PROGRAM MAIN
VAR
	init : BOOL;
	initSubstate : InitSubstate;
	axisPowerSubstate : AxisPowerSubstate; 
	solenoindExtendSubstate : SolenoindExtendSubstate;
	isInit, hasNext, isPower, isBackToInit : BOOL;
	applicationState  : ApplicationSubstate;
	
	axisModule : AxisModule(applicationState, InitSubstate := initSubstate, AxisPowerSubstate := solenoindExtendSubstate);
	pusherModule : PusherModule(applicationState);
END_VAR

IF NOT init THEN
	applicationState.AddSubstate(initSubstate);
	applicationState.AddSubstate(solenoindExtendSubstate);
	applicationState.AddSubstate(axisPowerSubstate);
	
	isInit := applicationState.CurrentState.IsEqual(initSubstate);
	hasNext := applicationState.MoveNext();
	hasNext := applicationState.MoveNext();
	isPower :=  applicationState.CurrentState.IsEqual(axisPowerSubstate);
	
	applicationState.Reset();
	isBackToInit :=  applicationState.CurrentState.IsEqual(initSubstate);

	init := TRUE;
	
	axisModule.Execute();
	pusherModule.Execute();
	
	isPower :=  applicationState.CurrentState.IsEqual(axisPowerSubstate);
	
END_IF

END_PROGRAM
